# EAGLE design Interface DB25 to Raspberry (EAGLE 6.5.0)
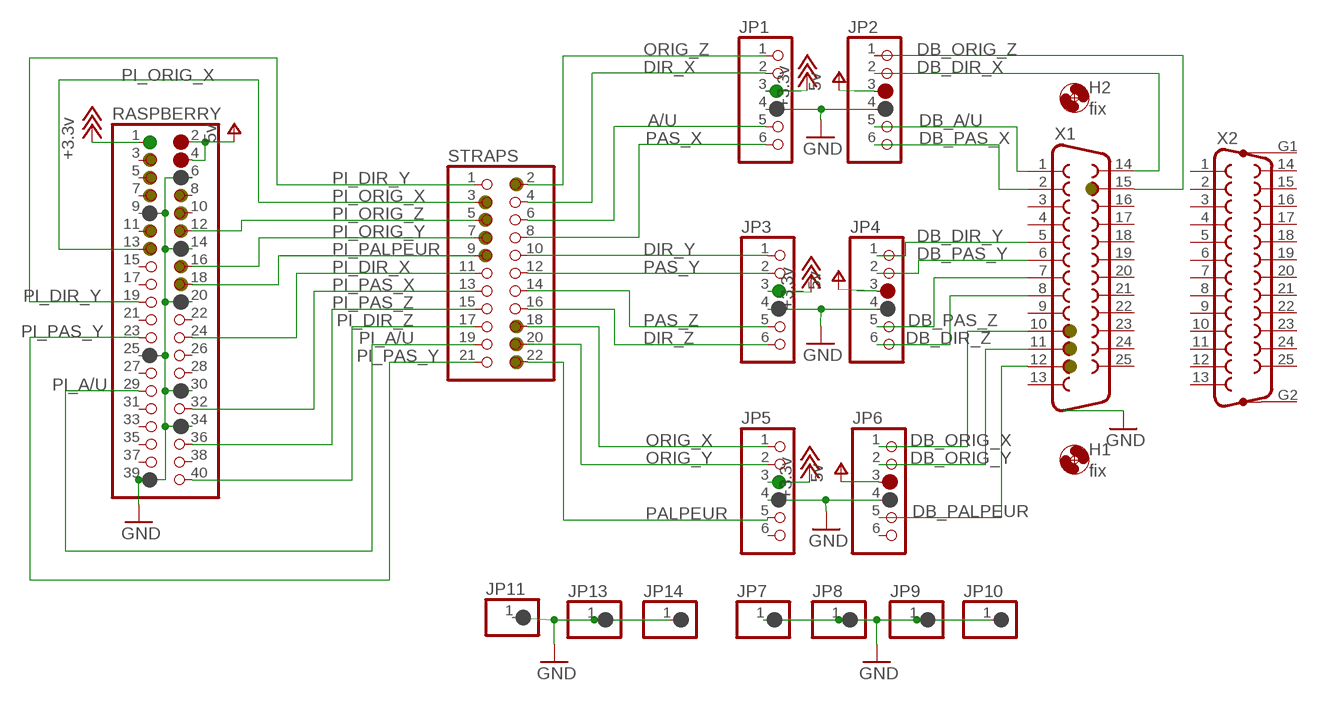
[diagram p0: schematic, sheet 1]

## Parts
H1  fix  MOUNT-HOLE3.6  [3,6]
H2  fix  MOUNT-HOLE3.6  [3,6]
JP1  PINHD-1X6  [1X06]
JP2  PINHD-1X6  [1X06]
JP3  PINHD-1X6  [1X06]
JP4  PINHD-1X6  [1X06]
JP5  PINHD-1X6  [1X06]
JP6  PINHD-1X6  [1X06]
JP7  PINHD-1X1  [1X01]
JP8  PINHD-1X1  [1X01]
JP9  PINHD-1X1  [1X01]
JP10  PINHD-1X1  [1X01]
JP11  PINHD-1X1  [1X01]
JP13  PINHD-1X1  [1X01]
JP14  PINHD-1X1  [1X01]
RASPBERRY  PINHD-2X20/OCT  [2X20]
STRAPS  PINHD-2X11  [2X11]
X1  F25HP  [F25HP]
X2  F25VP  [F25VP]

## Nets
+18V: JP1.3 JP3.3 JP5.3 RASPBERRY.1 ; supply symbol labelled +3.3v
A/U: JP1.5 STRAPS.6
DB_A/U: JP2.5 X1.1
DB_DIR_X: JP2.2 X1.14
DB_DIR_Y: JP4.1 X1.5
DB_DIR_Z: JP4.6 X1.8
DB_ORIG_X: JP6.1 X1.10
DB_ORIG_Y: JP6.2 X1.11
DB_ORIG_Z: JP2.1 X1.15
DB_PALPEUR: JP6.5 X1.12
DB_PAS_X: JP2.6 X1.2
DB_PAS_Y: JP4.2 X1.6
DB_PAS_Z: JP4.5 X1.7
DIR_X: JP1.2 STRAPS.4
DIR_Y: JP3.1 STRAPS.10
DIR_Z: JP3.6 STRAPS.16
GND: JP1.4 JP2.4 JP3.4 JP4.4 JP5.4 JP6.4 JP7.1 JP8.1 JP9.1 JP10.1 JP11.1 JP13.1 JP14.1 RASPBERRY.6 RASPBERRY.9 RASPBERRY.14 RASPBERRY.20 RASPBERRY.25 RASPBERRY.30 RASPBERRY.34 RASPBERRY.39
ORIG_X: JP5.1 STRAPS.18
ORIG_Y: JP5.2 STRAPS.20
ORIG_Z: JP1.1 STRAPS.2
PALPEUR: JP5.5 STRAPS.22
PAS_X: JP1.6 STRAPS.8
PAS_Y: JP3.2 STRAPS.12
PAS_Z: JP3.5 STRAPS.14
PI_A/U: RASPBERRY.29 STRAPS.19
PI_DIR_X: RASPBERRY.24 STRAPS.11
PI_DIR_Y: RASPBERRY.19 STRAPS.1
PI_DIR_Z: RASPBERRY.40 STRAPS.17
PI_ORIG_X: RASPBERRY.13 STRAPS.3
PI_ORIG_Y: RASPBERRY.16 STRAPS.7
PI_ORIG_Z: RASPBERRY.12 STRAPS.5
PI_PALPEUR: RASPBERRY.18 STRAPS.9
PI_PAS_X: RASPBERRY.32 STRAPS.13
PI_PAS_Y: RASPBERRY.23 STRAPS.21
PI_PAS_Z: RASPBERRY.36 STRAPS.15
V+: JP2.3 JP4.3 JP6.3 RASPBERRY.2 RASPBERRY.4 ; supply symbol labelled 5v
Unconnected: JP5.6 JP6.6 RASPBERRY.3 RASPBERRY.5 RASPBERRY.7 RASPBERRY.8 RASPBERRY.10 RASPBERRY.11 RASPBERRY.15 RASPBERRY.17 RASPBERRY.21 RASPBERRY.22 RASPBERRY.26 RASPBERRY.27 RASPBERRY.28 RASPBERRY.31 RASPBERRY.33 RASPBERRY.35 RASPBERRY.37 RASPBERRY.38 X1.3 X1.4 X1.9 X1.13 X1.16 X1.17 X1.18 X1.19 X1.20 X1.21 X1.22 X1.23 X1.24 X1.25 X2.1 X2.2 X2.3 X2.4 X2.5 X2.6 X2.7 X2.8 X2.9 X2.10 X2.11 X2.12 X2.13 X2.14 X2.15 X2.16 X2.17 X2.18 X2.19 X2.20 X2.21 X2.22 X2.23 X2.24 X2.25 X2.G1 X2.G2

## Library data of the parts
H1 H2 = holes:MOUNT-HOLE: MOUNTING HOLE with drill center marker
JP1-JP6 = pinhead:PINHD-1X6: PIN HEADER
JP7-JP11 JP13 JP14 = pinhead:PINHD-1X1: PIN HEADER
RASPBERRY = pinhead_v2:PINHD-2X20: PIN HEADER
STRAPS = pinhead:PINHD-2X11: PIN HEADER
X1 = con-subd:F25: SUB-D; OC_FARNELL: unknown; OC_NEWARK: unknown
X2 = con-subd:F25VP: SUB-D; OC_FARNELL: unknown; OC_NEWARK: unknown

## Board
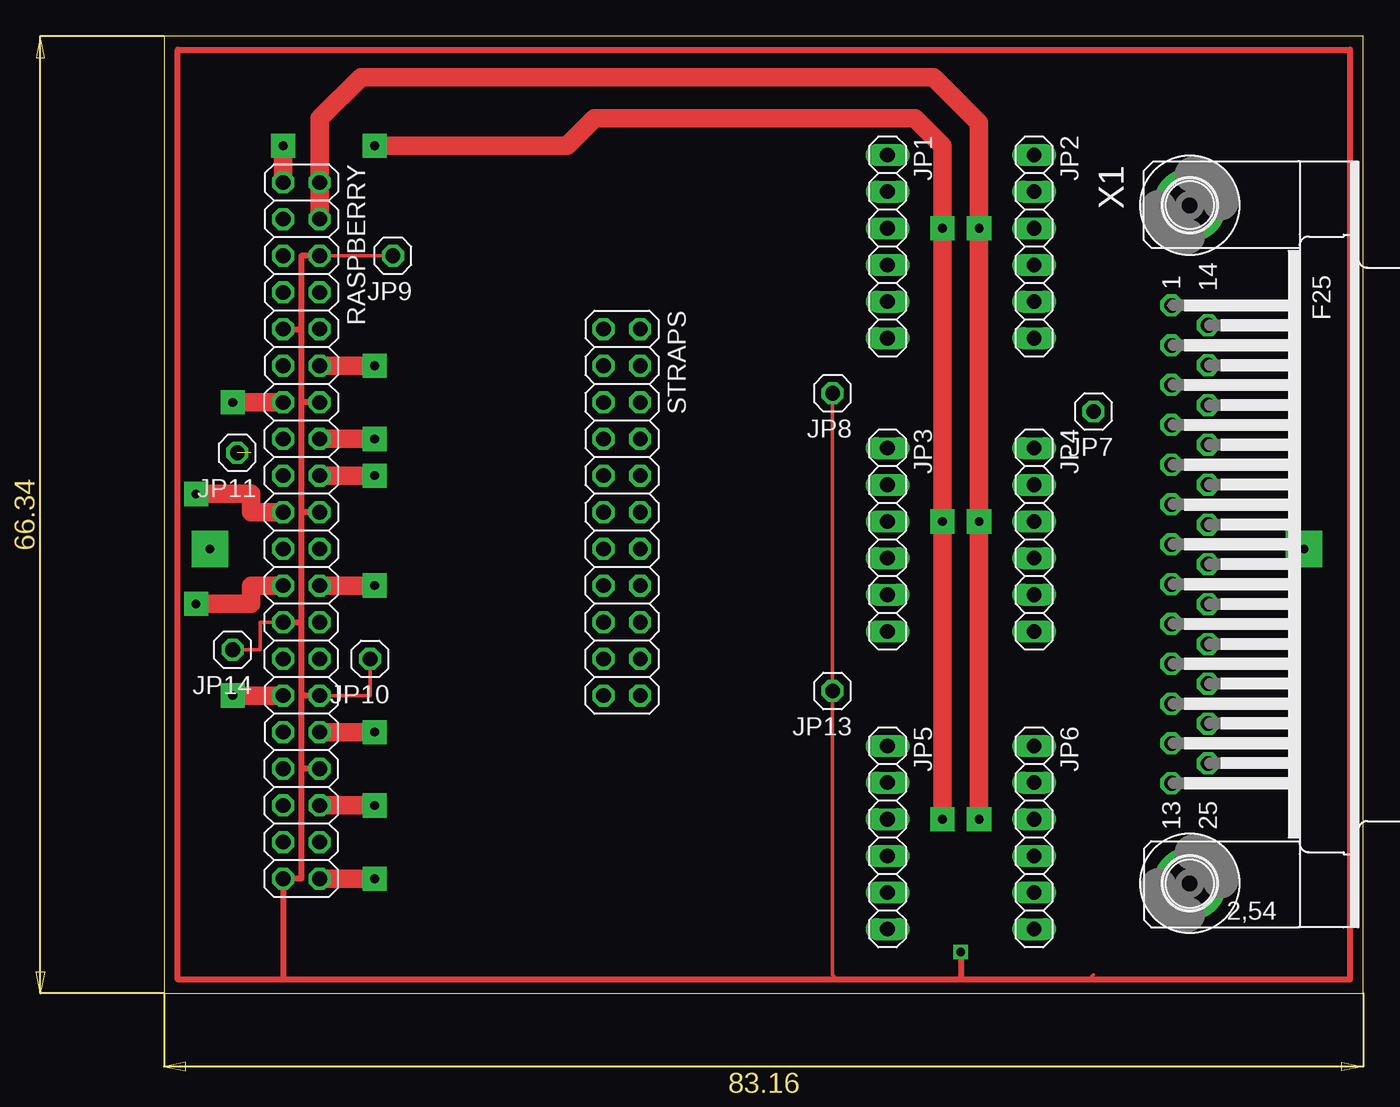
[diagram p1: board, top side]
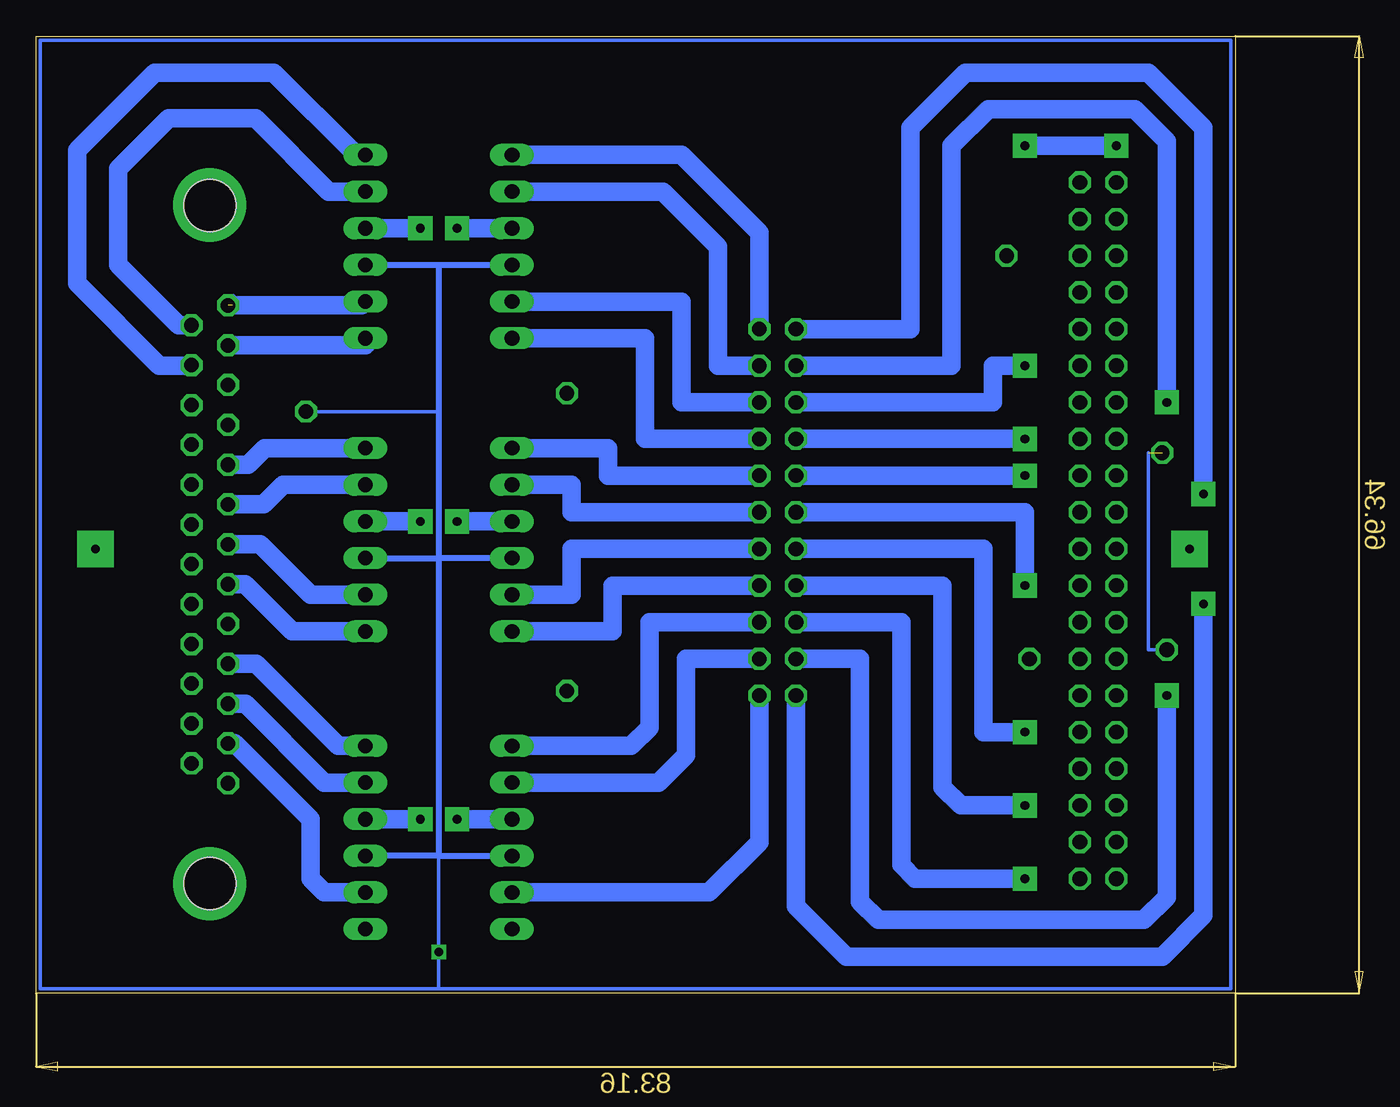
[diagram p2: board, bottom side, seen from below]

Size 92.04 x 71.72 mm. Coordinates in mm from the lower left corner, seen from the top.
Outline: 8.87,5.38 92.04,5.38 92.04,71.72 8.87,71.72 8.87,5.38
Copper layers (1*16): Top 0.035mm / dielectric 1.5mm / Bottom 0.035mm
Design rules "default": minimum track width 10mil, minimum drill 24mil, track to track 8mil, track to pad 8mil, pad to pad 8mil, via to via 8mil, smd to smd 8mil, copper to edge 40mil, drill to drill 8mil, minimum pad ring 10mil, minimum via ring 8mil, stop-mask expansion 4mil, vias tented up to drill 0mil, thermal gap 10mil

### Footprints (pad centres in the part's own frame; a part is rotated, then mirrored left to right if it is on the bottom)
3,6 = hole 3.6: 0,0
1X06 = drill 1.016 long: 1 -6.35,0; 2 -3.81,0; 3 -1.27,0; 4 1.27,0; 5 3.81,0; 6 6.35,0
1X01 = drill 1.016 octagon: 1 0,0
2X20 = drill 1.016 octagon: 1 -24.13,-1.27; 2 -24.13,1.27; 3 -21.59,-1.27; 4 -21.59,1.27; 5 -19.05,-1.27; 6 -19.05,1.27; 7 -16.51,-1.27; 8 -16.51,1.27; 9 -13.97,-1.27; 10 -13.97,1.27; 11 -11.43,-1.27; 12 -11.43,1.27; 13 -8.89,-1.27; 14 -8.89,1.27; 15 -6.35,-1.27; 16 -6.35,1.27; 17 -3.81,-1.27; 18 -3.81,1.27; 19 -1.27,-1.27; 20 -1.27,1.27; 21 1.27,-1.27; 22 1.27,1.27; 23 3.81,-1.27; 24 3.81,1.27; 25 6.35,-1.27; 26 6.35,1.27; 27 8.89,-1.27; 28 8.89,1.27; 29 11.43,-1.27; 30 11.43,1.27; 31 13.97,-1.27; 32 13.97,1.27; 33 16.51,-1.27; 34 16.51,1.27; 35 19.05,-1.27; 36 19.05,1.27; 37 21.59,-1.27; 38 21.59,1.27; 39 24.13,-1.27; 40 24.13,1.27
2X11 = drill 1.016 octagon: 1 -12.7,-1.27; 2 -12.7,1.27; 3 -10.16,-1.27; 4 -10.16,1.27; 5 -7.62,-1.27; 6 -7.62,1.27; 7 -5.08,-1.27; 8 -5.08,1.27; 9 -2.54,-1.27; 10 -2.54,1.27; 11 0,-1.27; 12 0,1.27; 13 2.54,-1.27; 14 2.54,1.27; 15 5.08,-1.27; 16 5.08,1.27; 17 7.62,-1.27; 18 7.62,1.27; 19 10.16,-1.27; 20 10.16,1.27; 21 12.7,-1.27; 22 12.7,1.27
F25HP = drill 1.016 octagon: 1 -16.561,-1.27; 2 -13.792,-1.27; 3 -11.049,-1.27; 4 -8.28,-1.27; 5 -5.512,-1.27; 6 -2.769,-1.27; 7 0,-1.27; 8 2.769,-1.27; 9 5.512,-1.27; 10 8.28,-1.27; 11 11.049,-1.27; 12 13.792,-1.27; 13 16.561,-1.27; 14 -15.189,1.27; 15 -12.421,1.27; 16 -9.652,1.27; 17 -6.909,1.27; 18 -4.14,1.27; 19 -1.372,1.27; 20 1.372,1.27; 21 4.14,1.27; 22 6.909,1.27; 23 9.652,1.27; 24 12.421,1.27; 25 15.189,1.27 | drill 3.302 pad 5.08: G1 -23.52,0; G2 23.52,0
F25VP = drill 1.016 octagon: 1 16.561,1.422; 2 13.792,1.422; 3 11.049,1.422; 4 8.28,1.422; 5 5.512,1.422; 6 2.769,1.422; 7 0,1.422; 8 -2.769,1.422; 9 -5.512,1.422; 10 -8.28,1.422; 11 -11.049,1.422; 12 -13.792,1.422; 13 -16.561,1.422; 14 15.189,-1.422; 15 12.421,-1.422; 16 9.652,-1.422; 17 6.909,-1.422; 18 4.14,-1.422; 19 1.372,-1.422; 20 -1.372,-1.422; 21 -4.14,-1.422; 22 -6.909,-1.422; 23 -9.652,-1.422; 24 -12.421,-1.422; 25 -15.189,-1.422 | drill 3.302 pad 5.08: G1 -23.52,0; G2 23.52,0

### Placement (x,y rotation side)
H1  79.99,59.99 0 top
H2  79.99,13 0 top
JP1  59.04,57.13 270 top
JP2  69.2,57.13 270 top
JP3  59.04,36.81 270 top
JP4  69.2,36.81 270 top
JP5  59.04,16.18 270 top
JP6  69.2,16.18 270 top
JP7  73.33,45.7 180 top
JP8  55.23,46.97 180 top
JP9  24.75,56.5 180 top
JP10  23.16,28.56 180 top
JP11  13.95,42.84 180 top
JP13  55.23,26.34 180 top
JP14  13.64,29.19 180 top
RASPBERRY  18.4,37.45 270 top
STRAPS  40.62,38.72 270 top
X1  79.99,36.5 270 top
X2  not placed on the board

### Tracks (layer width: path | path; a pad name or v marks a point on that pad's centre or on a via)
+18V  (via drill 0.6 pad 1.68)
  Top 1.27: v62.85,17.45 v62.85,38.08 v62.85,58.4 62.85,64.12 60.94,66.02 38.72,66.02 36.81,64.12 v23.48,64.12 | RASPBERRY.1 v17.13,64.12
  Bottom 1.27: v62.85,17.45 JP5.3 | JP3.3 v62.85,38.08 | JP1.3 v62.85,58.4 | v17.13,64.12 v23.48,64.12
A/U
  Bottom 1.27: JP1.5 47.29,53.32 47.29,46.34 STRAPS.6
DB_A/U  (1 unrouted)
  Bottom 0.406: 78.41,53.06 78.41,53.64 | 69.46,53.06 JP2.5
  Bottom 1.27: 78.41,53.06 69.46,53.06
DB_DIR_X
  Bottom 1.27: X1.14 82.16,51.68 86.34,55.86 86.34,62.53 82.85,66.02 76.82,66.02 71.74,60.94 JP2.2
DB_DIR_Y
  Bottom 1.27: X1.5 77.34,42.01 76.18,43.16 JP4.1
DB_DIR_Z
  Bottom 1.27: X1.8 77.54,33.73 74.28,30.46 JP4.6
DB_ORIG_X
  Bottom 1.27: X1.10 76.79,28.21 71.1,22.53 JP6.1
DB_ORIG_Y
  Bottom 1.27: X1.11 77.52,25.45 72.06,19.98 JP6.2
DB_ORIG_Z
  Bottom 0.406: 81.26,48.88 X1.15
  Bottom 1.27: 81.26,48.88 83.48,48.88 89.2,54.59 89.2,63.8 83.8,69.2 75.55,69.2 69.83,63.48 JP2.1
DB_PALPEUR
  Bottom 1.27: X1.12 78.27,22.7 73.01,17.45 73.01,13.32 72.06,12.37 JP6.5
DB_PAS_X
  Bottom 1.27: X1.2 69.2,50.29 JP2.6
DB_PAS_Y
  Bottom 1.27: X1.6 76.27,39.26 74.91,40.62 JP4.2
DB_PAS_Z
  Bottom 1.27: X1.7 76.5,36.5 73.01,33 JP4.5
DIR_X
  Bottom 1.27: STRAPS.4 44.75,48.88 44.75,57.13 48.56,60.94 JP1.2
DIR_Y
  Bottom 1.27: JP3.1 52.37,43.16 52.37,41.26 STRAPS.10
DIR_Z
  Bottom 1.27: JP3.6 52.05,30.46 52.05,33.64 STRAPS.16
GND  (via drill 0.6)  (1 unrouted)
  Top 0.254: 73.33,6.65 73.01,6.33 | 55.55,6.33 55.23,6.65 JP13.1 JP8.1 | JP10.1 23.16,26.02 RASPBERRY.30 | RASPBERRY.25 15.54,31.1 15.54,29.19 JP14.1 | RASPBERRY.6 JP9.1
  Top 0.406: 64.12,6.33 73.01,6.33 91.11,6.33 91.11,70.79 9.83,70.79 9.83,6.33 17.13,6.33 | 64.12,6.33 55.55,6.33 17.13,6.33 | v64.12,8.24 64.12,6.33 | RASPBERRY.6 18.4,56.5 18.4,51.42 | 18.4,51.42 18.4,46.34 | 18.4,46.34 18.4,38.72 | 18.4,38.72 18.4,31.1 | 18.4,31.1 18.4,26.02 | 18.4,26.02 18.4,20.94 | 18.4,20.94 18.4,13.32 RASPBERRY.39 17.13,6.33 | RASPBERRY.34 18.4,20.94 | RASPBERRY.30 18.4,26.02 | RASPBERRY.25 18.4,31.1 | RASPBERRY.20 18.4,38.72 | RASPBERRY.14 18.4,46.34 | RASPBERRY.9 18.4,51.42
  Bottom 0.254: 64.12,5.7 91.74,5.7 91.74,71.42 9.19,71.42 9.19,5.7 64.12,5.7 | 64.12,14.9 v64.12,8.24 64.12,5.7 | JP14.1 14.91,29.19 14.91,42.84 | JP7.1 64.12,45.7
  Bottom 0.406: JP4.4 64.12,35.54 | 64.12,14.9 JP5.4 | JP3.4 64.12,35.54 | 64.12,35.54 64.12,14.9 | 64.12,55.86 64.12,45.7 64.12,35.54 | JP2.4 64.12,55.86 | 64.12,55.86 JP1.4 | 64.12,14.9 JP6.4
N$1  (via drill 0.6 pad 2.54)
  other vias: 87.93,36.18
N$3  (via drill 0.6 pad 2.54)
  other vias: 12.05,36.18
ORIG_X
  Bottom 1.27: STRAPS.18 49.51,31.1 49.51,23.79 50.78,22.53 JP5.1
ORIG_Y
  Bottom 1.27: STRAPS.20 46.97,28.56 46.97,21.89 48.88,19.98 JP5.2
ORIG_Z
  Bottom 1.27: JP1.1 47.29,63.48 41.89,58.08 STRAPS.2
PALPEUR
  Bottom 1.27: JP5.5 45.39,12.37 41.89,15.86 STRAPS.22
PAS_X
  Bottom 1.27: JP1.6 49.83,50.78 49.83,43.8 STRAPS.8
PAS_Y
  Bottom 1.27: JP3.2 54.91,40.62 54.91,38.72 STRAPS.12
PAS_Z
  Bottom 1.27: JP3.5 54.91,33 54.91,36.18 STRAPS.14
PI_A/U  (via drill 0.6 pad 1.68)
  Top 1.27: v13.64,26.02 RASPBERRY.29
  Bottom 1.27: STRAPS.19 34.91,28.56 34.91,11.73 33.64,10.46 15.22,10.46 13.64,12.05 v13.64,26.02
PI_DIR_X  (via drill 0.6 pad 1.68)
  Top 1.27: v23.48,33.64 RASPBERRY.24
  Bottom 1.27: v23.48,33.64 23.48,38.72 STRAPS.11
PI_DIR_Y  (via drill 0.6 pad 1.68)
  Top 1.27: v11.1,39.99 14.91,39.99 14.91,38.72 RASPBERRY.19
  Bottom 1.27: STRAPS.1 31.42,51.42 31.42,65.39 27.61,69.2 14.91,69.2 11.1,65.39 v11.1,39.99
PI_DIR_Z  (via drill 0.6 pad 1.68)
  Top 1.27: v23.48,13.32 RASPBERRY.40
  Bottom 1.27: STRAPS.17 32.05,31.1 32.05,14.27 31.1,13.32 v23.48,13.32
PI_ORIG_X  (via drill 0.6 pad 1.68)
  Top 1.27: v13.64,46.34 RASPBERRY.13
  Bottom 1.27: STRAPS.3 28.56,48.88 28.56,64.12 26.02,66.66 15.86,66.66 13.64,64.44 v13.64,46.34
PI_ORIG_Y  (via drill 0.6 pad 1.68)
  Top 1.27: v23.48,43.8 RASPBERRY.16
  Bottom 1.27: STRAPS.7 v23.48,43.8
PI_ORIG_Z  (via drill 0.6 pad 1.68)
  Top 1.27: v23.48,48.88 RASPBERRY.12
  Bottom 1.27: STRAPS.5 25.7,46.34 25.7,48.88 v23.48,48.88
PI_PALPEUR  (via drill 0.6 pad 1.68)
  Top 1.27: RASPBERRY.18 v23.48,41.26
  Bottom 1.27: v23.48,41.26 STRAPS.9
PI_PAS_X  (via drill 0.6 pad 1.68)
  Top 1.27: v23.48,23.48 RASPBERRY.32
  Bottom 1.27: STRAPS.13 26.34,36.18 26.34,23.48 v23.48,23.48
PI_PAS_Y  (via drill 0.6 pad 1.68)
  Top 1.27: v11.1,32.37 14.91,32.37 14.91,33.64 RASPBERRY.23
  Bottom 1.27: STRAPS.21 39.35,11.41 35.86,7.92 13.95,7.92 11.1,10.78 v11.1,32.37
PI_PAS_Z  (via drill 0.6 pad 1.68)
  Top 1.27: v23.48,18.4 RASPBERRY.36
  Bottom 1.27: STRAPS.15 29.19,33.64 29.19,19.67 27.92,18.4 v23.48,18.4
V+  (via drill 0.6 pad 1.68)
  Top 1.27: v65.39,17.45 v65.39,38.08 v65.39,58.4 65.39,65.71 62.21,68.88 22.53,68.88 19.67,66.02 RASPBERRY.2 RASPBERRY.4
  Bottom 1.27: v65.39,17.45 JP6.3 | JP4.3 v65.39,38.08 | JP2.3 v65.39,58.4

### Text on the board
Document: 5v | 5v | 3.3v | 3.3v | A/U | orig_Z | dir_Y | pas_X | dir_X | dir_X | orig_X | A/U | orig_Z | orig_Z | pas_X | orig_Y | dir_Y | dir_Y | palpeur | pas_Y | pas_Y | dir_X | pas_Z | pas_Z | pas_X | dir_Z | dir_Z | pas_Z | orig_X | dir_Z | orig_Y | orig_X | A/U | palpeur | pas_Y | orig_Y | palpeur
